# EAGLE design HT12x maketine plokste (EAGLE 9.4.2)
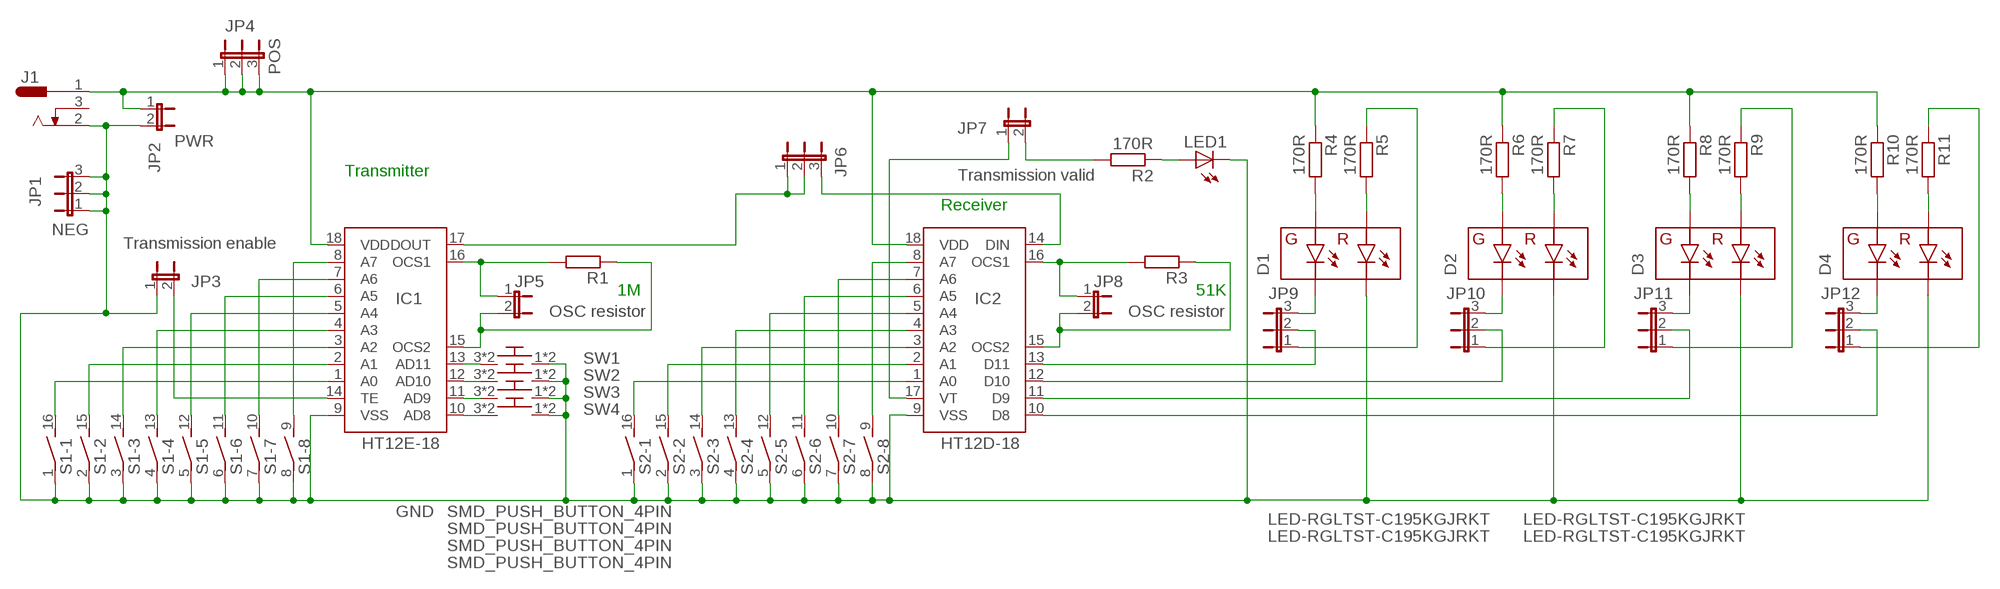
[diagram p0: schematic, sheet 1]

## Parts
D1  LED-RGLTST-C195KGJRKT  [LTST-C195KGJRKT]
D2  LED-RGLTST-C195KGJRKT  [LTST-C195KGJRKT]
D3  LED-RGLTST-C195KGJRKT  [LTST-C195KGJRKT]
D4  LED-RGLTST-C195KGJRKT  [LTST-C195KGJRKT]
IC1  HT12E-18  [DIP-18]
IC2  HT12D-18  [DIP-18]
J1  DC_JACK  [0.7X3MM]
JP1  NEG  JP2E  [JP2]
JP2  PWR  JP1E  [JP1]
JP3  Transmission enable  JP1E  [JP1]
JP4  POS  JP2E  [JP2]
JP5  OSC resistor  JP1E  [JP1]
JP6  JP2E  [JP2]
JP7  Transmission valid  JP1E  [JP1]
JP8  OSC resistor  JP1E  [JP1]
JP9  JP2E  [JP2]
JP10  JP2E  [JP2]
JP11  JP2E  [JP2]
JP12  JP2E  [JP2]
LED1  LED5MM  [LED5MM]
R1  R-EU_R0805W  [R0805W]
R2  170R  R-EU_R0805W  [R0805W]
R3  R-EU_R0805W  [R0805W]
R4  170R  R-EU_R0805W  [R0805W]
R5  170R  R-EU_R0805W  [R0805W]
R6  170R  R-EU_R0805W  [R0805W]
R7  170R  R-EU_R0805W  [R0805W]
R8  170R  R-EU_R0805W  [R0805W]
R9  170R  R-EU_R0805W  [R0805W]
R10  170R  R-EU_R0805W  [R0805W]
R11  170R  R-EU_R0805W  [R0805W]
S1  DIP08S  [DIP08S]
S2  DIP08S  [DIP08S]
SW1  SMD_PUSH_BUTTON_4PIN  [SMD_PUSH_BUTTON_4PIN]
SW2  SMD_PUSH_BUTTON_4PIN  [SMD_PUSH_BUTTON_4PIN]
SW3  SMD_PUSH_BUTTON_4PIN  [SMD_PUSH_BUTTON_4PIN]
SW4  SMD_PUSH_BUTTON_4PIN  [SMD_PUSH_BUTTON_4PIN]

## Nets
GND: D1.P$4(RC) D2.P$4(RC) D3.P$4(RC) D4.P$4(RC) IC1.9(VSS) IC2.9(VSS) J1.2 JP1.1 JP1.2 JP1.3 JP2.2 JP3.1 LED1.K(C) S1.1 S1.2 S1.3 S1.4 S1.5 S1.6 S1.7 S1.8 S2.1 S2.2 S2.3 S2.4 S2.5 S2.6 S2.7 S2.8 SW1.1 SW1.2 SW2.1 SW2.2 SW3.1 SW3.2 SW4.1 SW4.2
N$1: D1.P$3(GC) JP9.3
N$2: IC2.1(A0) S2.16
N$3: IC1.1(A0) S1.16
N$4: IC1.2(A1) S1.15
N$5: IC1.3(A2) S1.14
N$6: IC1.4(A3) S1.13
N$7: IC1.5(A4) S1.12
N$8: IC1.6(A5) S1.11
N$9: IC1.7(A6) S1.10
N$10: IC1.8(A7) S1.9
N$11: IC1.13(AD11) SW1.3 SW1.4
N$12: IC1.12(AD10) SW2.3 SW2.4
N$13: IC1.11(AD9) SW3.3 SW3.4
N$14: IC1.10(AD8) SW4.3 SW4.4
N$15: IC2.2(A1) S2.15
N$16: IC2.3(A2) S2.14
N$17: IC2.4(A3) S2.13
N$18: IC2.5(A4) S2.12
N$19: IC2.6(A5) S2.11
N$20: IC2.7(A6) S2.10
N$21: IC2.8(A7) S2.9
N$22: IC2.12(D10) JP10.2
N$23: D2.P$3(GC) JP10.3
N$24: JP10.1 R7.1
N$25: IC2.13(D11) JP9.2
N$26: D1.P$1(GA) R4.2
N$27: D2.P$1(GA) R6.2
N$28: D2.P$2(RA) R7.2
N$29: IC1.18(VDD) IC2.18(VDD) J1.1 JP2.1 JP4.1 JP4.2 JP4.3 R4.1 R6.1 R8.1 R10.1
N$30: IC2.11(D9) JP11.2
N$31: D3.P$3(GC) JP11.3
N$32: JP11.1 R9.1
N$34: IC1.17(DOUT) JP6.1 JP6.2
N$35: IC2.14(DIN) JP6.3
N$36: IC1.15(OCS2) JP5.2 R1.1
N$37: IC1.16(OCS1) JP5.1 R1.2
N$38: IC1.14(TE) JP3.2
N$39: IC2.15(OCS2) JP8.2 R3.1
N$40: IC2.16(OCS1) JP8.1 R3.2
N$41: IC2.17(VT) JP7.1
N$42: LED1.A R2.1
N$43: JP7.2 R2.2
N$44: JP9.1 R5.1
N$45: D1.P$2(RA) R5.2
N$46: D3.P$1(GA) R8.2
N$47: D3.P$2(RA) R9.2
N$49: IC2.10(D8) JP12.2
N$50: D4.P$3(GC) JP12.3
N$51: JP12.1 R11.1
N$52: D4.P$1(GA) R10.2
N$53: D4.P$2(RA) R11.2
Unconnected: J1.3

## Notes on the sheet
- Transmitter
- Receiver
- 1M | 51K

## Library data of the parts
D1-D4 = SparkFun-LED:LED-RG; PROD_ID: DIO-12140
IC1 = 433-869:HT12E: Features Operating voltage 2.4V~5V for the HT12A 2.4V~12V for the HT12E Low power and high noise immunity CMOS technology Low standby current: 0.1A (typ.) at VDD=5V HT12A with a 38kHz carrier for infrared transmission medium Minimum transmission word Four words for the HT12E One word for the HT12A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
IC2 = 433-869:HT12D: Features Operating voltage: 2.4V~12V Low power and high noise immunity CMOS technology Low standby current Capable of decoding 12 bits of information Binary address setting Received codes are checked 3 times Address/Data number combination HT12D: 8 address bits and 4 data bits HT12F: 12 address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
J1 = Wurth DC power jack:DC_JACK: DC Power Jack THT Right Angled Low Profile(2.8) Characteristics MATERIAL PROPERTIES Color Black Insulator Material PA66 Contact Material Copper Alloy Contact Type Stamped Center Pin Plating Gold Tip Spring Material Tin Shunt Terminal Plating Tin Cover Material Brass Cover Plating Tin OTHER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
JP1 JP4 JP6 JP9-JP12 = jumper:JP2E: JUMPER
JP2 JP3 JP5 JP7 JP8 = jumper:JP1E: JUMPER
LED1 = led:LED: LED
R1-R11 = rcl:R-EU_: RESISTOR, European symbol
S1 S2 = switch-dil:DIP08S: DIL/CODE SWITCH; OC_FARNELL: unknown; OC_NEWARK: unknown
SW1-SW4 = SMD push button:SMD_PUSH_BUTTON_4PIN: SMD push button, 4 pins.

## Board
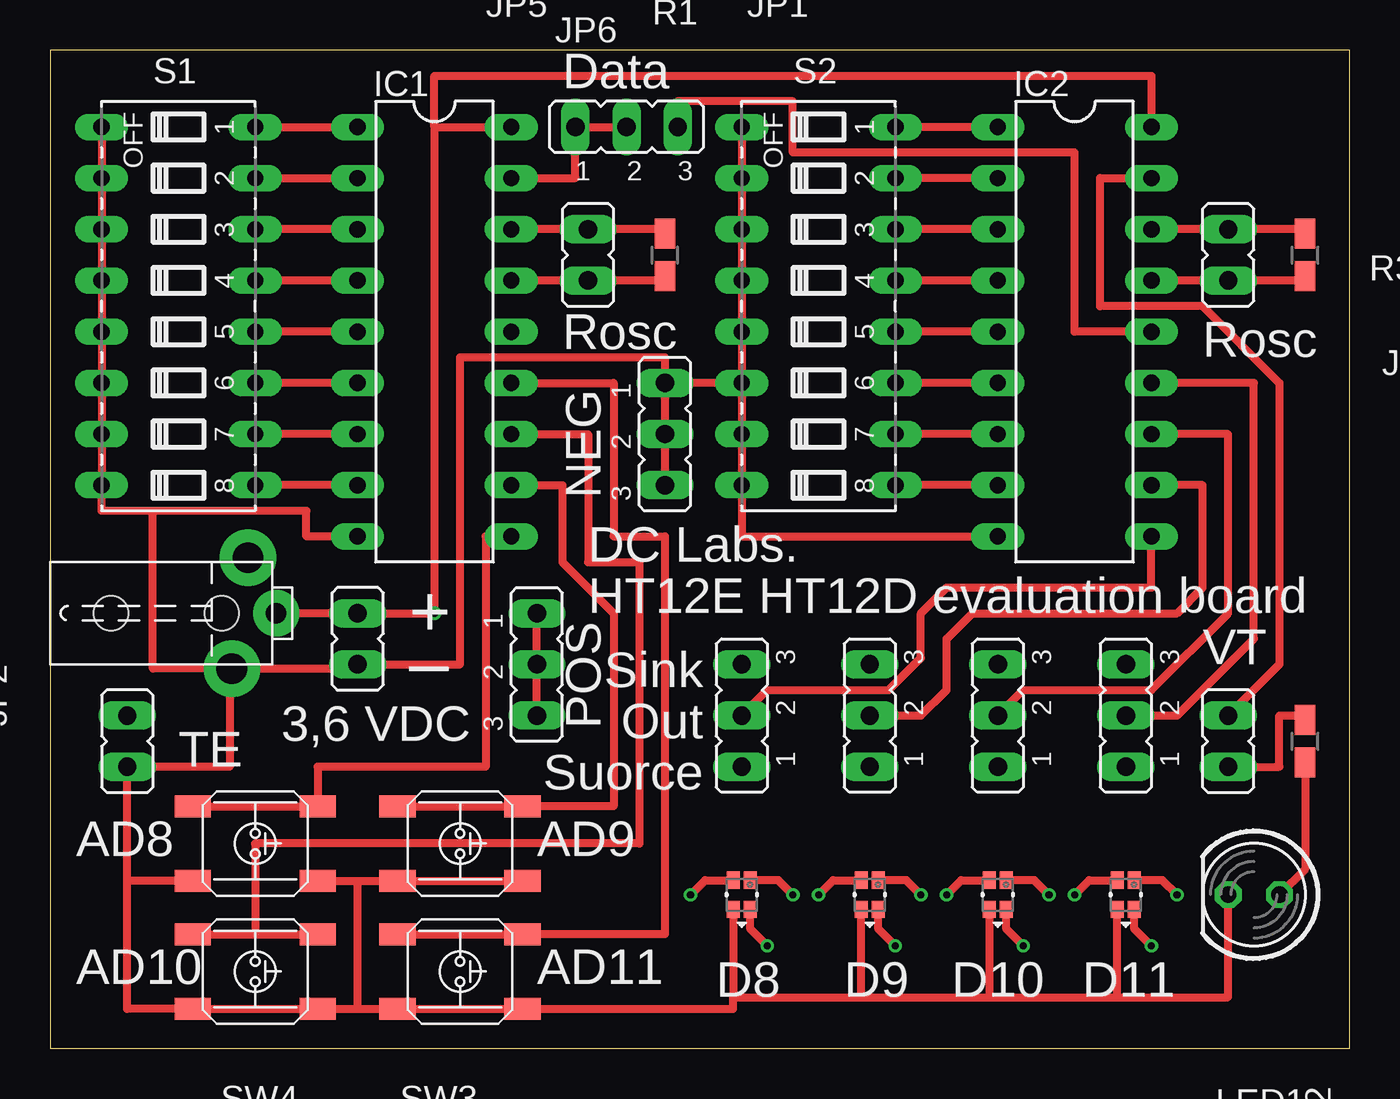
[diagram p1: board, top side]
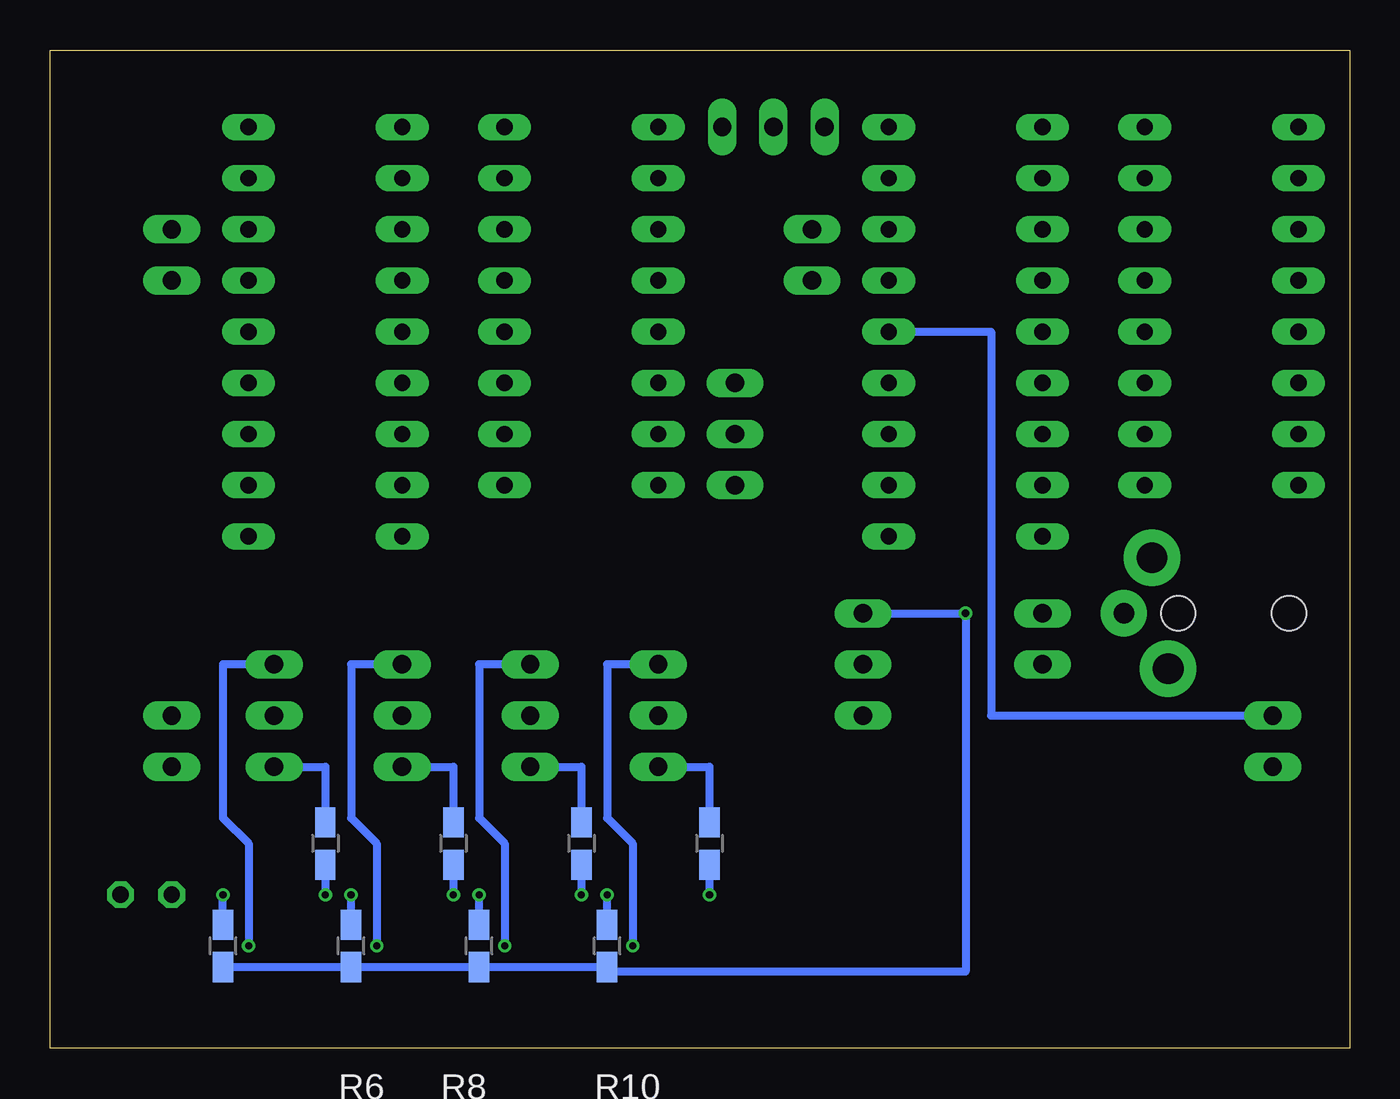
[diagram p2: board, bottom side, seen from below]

Size 64.44 x 49.52 mm. Coordinates in mm from the lower left corner, seen from the top.
Outline: 0,0 64.44,0 64.44,49.52 0,49.52 0,0
Copper layers (1*16): Top 0.035mm / dielectric 1.5mm / Bottom 0.035mm
Design rules "SeeedStudio_2layer_DRU_no_angle_20140221": minimum track width 6mil, minimum drill 12mil, track to track 6mil, track to pad 6mil, pad to pad 6mil, via to via 6mil, smd to smd 0mil, copper to edge 10mil, drill to drill 10mil, minimum pad ring 10mil, minimum via ring 6mil, stop-mask expansion 2mil, vias tented up to drill 100mil, thermal gap 10mil

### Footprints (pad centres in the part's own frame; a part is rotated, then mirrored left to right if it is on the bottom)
LTST-C195KGJRKT = smd 0.65 x 0.85: P$1 0.425,0.725; P$2 -0.425,0.725; P$3 0.425,-0.725; P$4 -0.425,-0.725
DIP-18 = drill 0.813 long: 1 -3.81,10.16; 2 -3.81,7.62; 3 -3.81,5.08; 4 -3.81,2.54; 5 -3.81,0; 6 -3.81,-2.54; 7 -3.81,-5.08; 8 -3.81,-7.62; 9 -3.81,-10.16; 10 3.81,-10.16; 11 3.81,-7.62; 12 3.81,-5.08; 13 3.81,-2.54; 14 3.81,0; 15 3.81,2.54; 16 3.81,5.08; 17 3.81,7.62; 18 3.81,10.16
0.7X3MM = drill 1.016 pad 2.286: 1 0,11.2 | drill 1.524 pad 2.794: 2 2.75,9; 3 -2.75,9.8 | hole 1.7: 0,3; 0,8.5
JP2 = drill 0.914 long: 1 -2.54,0; 2 0,0; 3 2.54,0
JP1 = drill 0.914 long: 1 0,-1.27; 2 0,1.27
LED5MM = drill 0.813 octagon: A -1.27,0; K 1.27,0
R0805W = smd 1.5 x 1: 1 -1.052,0; 2 1.052,0
DIP08S = drill 0.813 long: 1 -8.89,-3.81; 2 -6.35,-3.81; 3 -3.81,-3.81; 4 -1.27,-3.81; 5 1.27,-3.81; 6 3.81,-3.81; 7 6.35,-3.81; 8 8.89,-3.81; 9 8.89,3.81; 10 6.35,3.81; 11 3.81,3.81; 12 1.27,3.81; 13 -1.27,3.81; 14 -3.81,3.81; 15 -6.35,3.81; 16 -8.89,3.81
SMD_PUSH_BUTTON_4PIN = smd 1.8 x 1.1: 1 -3.1,1.85; 2 3.1,1.85; 3 -3.1,-1.85; 4 3.1,-1.85

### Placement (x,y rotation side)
D1  53.34,7.62 0 top
D2  46.99,7.62 0 top
D3  40.64,7.62 0 top
D4  34.29,7.62 0 top
IC1  19.05,35.56 0 top
IC2  50.8,35.56 0 top
J1  0,21.59 270 top
JP1  30.48,30.48 270 top
JP2  15.24,20.32 180 top
JP3  3.81,15.24 0 top
JP4  24.13,19.05 270 top
JP5  26.67,39.37 180 top
JP6  28.57,45.72 0 top
JP7  58.42,15.24 180 top
JP8  58.42,39.37 180 top
JP9  53.34,16.51 90 top
JP10  46.99,16.51 90 top
JP11  40.64,16.51 90 top
JP12  34.29,16.51 90 top
LED1  59.69,7.62 180 top
R1  30.48,39.37 90 top
R2  62.23,15.24 90 top
R3  62.23,39.37 90 top
R4  55.88,5.08 90 bottom
R5  50.8,10.16 270 bottom
R6  49.53,5.08 90 bottom
R7  44.45,10.16 270 bottom
R8  43.18,5.08 90 bottom
R9  38.1,10.16 270 bottom
R10  36.83,5.08 90 bottom
R11  31.75,10.16 270 bottom
S1  6.35,36.83 270 top
S2  38.1,36.83 270 top
SW1  20.32,3.81 180 top
SW2  10.16,3.81 180 top
SW3  20.32,10.16 180 top
SW4  10.16,10.16 180 top

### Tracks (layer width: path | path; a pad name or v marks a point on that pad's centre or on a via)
GND
  Top 0.406: S1.1 S1.2 S1.3 S1.4 S1.5 S1.6 S1.7 S1.8 2.54,26.67 5.08,26.67 | S2.1 S2.2 S2.3 S2.4 S2.5 S2.6 | S2.6 S2.7 S2.8 34.29,25.4 IC2.9 | D4.P$4 33.87,2.54 | 40.22,2.54 D3.P$4 | 33.87,2.54 40.22,2.54 | D2.P$4 46.56,2.54 | 40.22,2.54 46.56,2.54 | 46.56,2.54 52.91,2.54 | 52.91,2.54 D1.P$4 | 52.91,2.54 58.42,2.54 LED1.K | SW4.1 15.24,8.31 | 15.24,8.31 SW3.2 SW3.1 | 15.24,1.96 SW2.1 SW2.2 3.81,1.96 3.81,8.31 | 15.24,1.96 SW1.2 SW1.1 33.87,1.96 33.87,2.54 | 15.24,1.96 15.24,8.31 | 3.81,8.31 JP3.1 8.89,13.97 8.89,18.84 J1.2 | SW4.2 3.81,8.31 | J1.2 15.24,18.84 JP2.2 20.32,19.05 20.32,34.29 30.48,34.29 JP1.1 | J1.2 5.08,18.84 5.08,26.67 | IC1.9 12.7,25.4 12.7,26.67 5.08,26.67 | S2.6 JP1.1 | JP1.1 JP1.2 JP1.3
N$1  (via drill 0.35)
  Top 0.406: v54.61,5.08 53.77,5.92 D1.P$3
  Bottom 0.406: JP9.3 55.88,19.05 55.88,11.43 54.61,10.16 v54.61,5.08
N$2
  Top 0.406: IC2.1 46.33,45.72 42.57,45.72 S2.16
N$3
  Top 0.406: S1.16 IC1.1
N$4
  Top 0.406: S1.15 IC1.2
N$5
  Top 0.406: IC1.3 14.58,40.64 10.82,40.64 S1.14
N$6
  Top 0.406: IC1.4 14.58,38.1 10.82,38.1 S1.13
N$7
  Top 0.406: IC1.5 14.58,35.56 10.82,35.56 S1.12
N$8
  Top 0.406: IC1.6 14.58,33.02 10.82,33.02 S1.11
N$9
  Top 0.406: IC1.7 14.58,30.48 10.82,30.48 S1.10
N$10
  Top 0.406: IC1.8 14.58,27.94 10.82,27.94 S1.9
N$11
  Top 0.406: SW1.4 SW1.3 30.48,5.66 30.48,25.4 27.94,25.4 27.94,33.02 IC1.13
N$12
  Top 0.406: SW2.4 10.16,5.66 | 10.16,5.66 SW2.3 | IC1.12 26.67,30.48 26.67,24.13 29.21,24.13 29.21,10.16 10.16,10.16 10.16,5.66
N$13
  Top 0.406: SW3.4 SW3.3 27.94,12.01 27.94,21.59 25.4,24.13 25.4,27.94 IC1.11
N$14
  Top 0.406: SW4.4 SW4.3 13.26,13.97 21.59,13.97 21.59,25.4 IC1.10
N$15
  Top 0.406: IC2.2 46.33,43.18 42.57,43.18 S2.15
N$16
  Top 0.406: IC2.3 46.33,40.64 42.57,40.64 S2.14
N$17
  Top 0.406: IC2.4 46.33,38.1 42.57,38.1 S2.13
N$18
  Top 0.406: IC2.5 46.33,35.56 42.57,35.56 S2.12
N$19
  Top 0.406: IC2.6 46.33,33.02 42.57,33.02 S2.11
N$20
  Top 0.406: IC2.7 46.33,30.48 42.57,30.48 S2.10
N$21
  Top 0.406: IC2.8 46.33,27.94 42.57,27.94 S2.9
N$22
  Top 0.406: JP10.2 48.26,17.78 54.61,17.78 58.42,21.59 58.42,30.48 IC2.12
N$23  (via drill 0.35)
  Top 0.406: v48.26,5.08 47.41,5.92 D2.P$3
  Bottom 0.406: JP10.3 49.53,19.05 49.53,11.43 48.26,10.16 v48.26,5.08
N$24
  Bottom 0.406: JP10.1 44.45,13.97 R7.1
N$25
  Top 0.406: JP9.2 55.88,16.51 59.69,20.32 59.69,33.02 IC2.13
N$26  (via drill 0.35)
  Top 0.406: v55.88,7.62 55.16,8.35 D1.P$1
  Bottom 0.406: R4.2 v55.88,7.62
N$27  (via drill 0.35)
  Top 0.406: v49.53,7.62 48.8,8.35 D2.P$1
  Bottom 0.406: R6.2 v49.53,7.62
N$28  (via drill 0.35)
  Top 0.406: v44.45,7.62 45.17,8.35 D2.P$2
  Bottom 0.406: R7.2 v44.45,7.62
N$29  (via drill 0.35)
  Top 0.406: J1.1 JP2.1 v19.05,21.59 19.05,45.72 | 19.05,45.72 IC1.18 | 19.05,45.72 19.05,48.26 54.61,48.26 IC2.18 | JP4.3 JP4.2 JP4.1
  Bottom 0.406: R4.1 R6.1 R8.1 R10.1 36.83,3.81 19.05,3.81 v19.05,21.59 JP4.1
N$30
  Top 0.406: JP11.2 43.18,16.51 44.45,17.78 44.45,20.32 45.72,21.59 55.88,21.59 57.15,22.86 57.15,27.94 IC2.11
N$31  (via drill 0.35)
  Top 0.406: v41.91,5.08 41.06,5.92 D3.P$3
  Bottom 0.406: JP11.3 43.18,19.05 43.18,11.43 41.91,10.16 v41.91,5.08
N$32
  Bottom 0.406: JP11.1 38.1,13.97 R9.1
N$34
  Top 0.406: IC1.17 26.04,43.18 JP6.1 JP6.2
N$35
  Top 0.406: IC2.14 50.8,35.56 50.8,44.45 36.83,44.45 36.83,46.99 31.11,46.99 JP6.3
N$36
  Top 0.406: IC1.15 23.52,38.1 25.96,38.1 JP5.2 27.38,38.1 30.26,38.1 R1.1
N$37
  Top 0.406: IC1.16 23.52,40.64 25.96,40.64 JP5.1 27.38,40.64 30.26,40.64 R1.2
N$38
  Bottom 0.406: IC1.14 17.78,35.56 17.78,16.51 JP3.2
N$39
  Top 0.406: IC2.15 55.27,38.1 57.71,38.1 JP8.2 59.13,38.1 62.01,38.1 R3.1
N$40
  Top 0.406: IC2.16 55.27,40.64 57.71,40.64 JP8.1 59.13,40.64 62.01,40.64 R3.2
N$41
  Top 0.406: JP7.1 60.96,19.05 60.96,33.02 57.15,36.83 52.07,36.83 52.07,43.18 IC2.17
N$42
  Top 0.406: R2.1 62.23,8.89 LED1.A
N$43
  Top 0.406: JP7.2 60.96,13.97 60.96,16.51 62.01,16.51 R2.2
N$44
  Bottom 0.406: JP9.1 50.8,13.97 R5.1
N$45  (via drill 0.35)
  Top 0.406: v50.8,7.62 51.52,8.35 D1.P$2
  Bottom 0.406: R5.2 v50.8,7.62
N$46  (via drill 0.35)
  Top 0.406: v43.18,7.62 42.45,8.35 D3.P$1
  Bottom 0.406: R8.2 v43.18,7.62
N$47  (via drill 0.35)
  Top 0.406: v38.1,7.62 38.83,8.35 D3.P$2
  Bottom 0.406: R9.2 v38.1,7.62
N$49
  Top 0.406: JP12.2 35.56,17.78 41.59,17.78 43.18,19.37 43.18,21.59 44.45,22.86 54.61,22.86 IC2.10
N$50  (via drill 0.35)
  Top 0.406: v35.56,5.08 34.72,5.92 D4.P$3
  Bottom 0.406: JP12.3 36.83,19.05 36.83,11.43 35.56,10.16 v35.56,5.08
N$51
  Bottom 0.406: JP12.1 31.75,13.97 R11.1
N$52  (via drill 0.35)
  Top 0.406: v36.83,7.62 36.1,8.35 D4.P$1
  Bottom 0.406: R10.2 v36.83,7.62
N$53  (via drill 0.35)
  Top 0.406: v31.75,7.62 32.48,8.35 D4.P$2
  Bottom 0.406: R11.2 v31.75,7.62

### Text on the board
tNames: Data | Rosc | Rosc | NEG | DC Labs. | HT12E HT12D evaluation board | + | Sink | VT | ‒ | Out | POS | 3,6 VDC | Suorce | TE | AD8 | AD9 | AD10 | AD11 | D8 | D9 | D10 | D11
